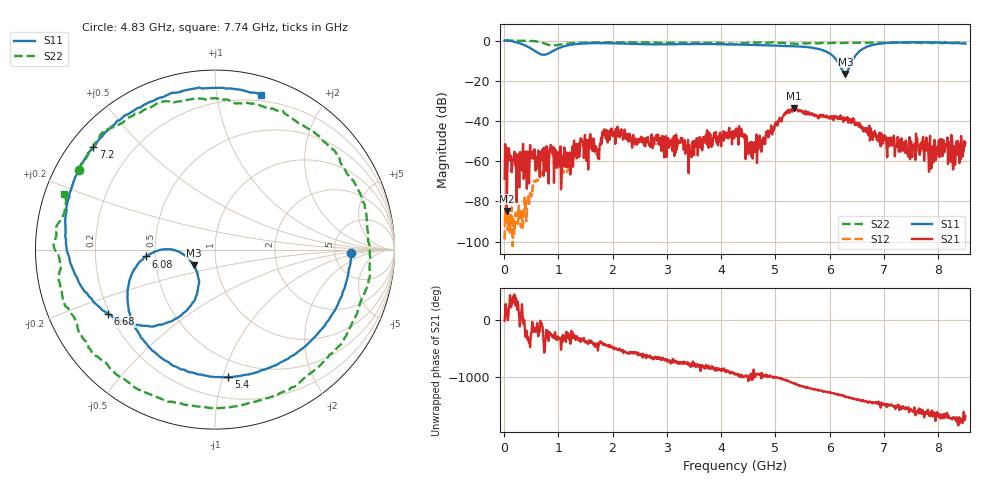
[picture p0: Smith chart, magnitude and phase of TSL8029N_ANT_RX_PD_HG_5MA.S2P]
!Agilent Technologies,E5071C,MY46523237,B.13.01
!Date: Wed Oct 18 11:31:03 2023
!Data & Calibration Information:
!Freq	S11:SOLT2(ON)	S21:SOLT2(ON)	S12:SOLT2(ON)	S22:SOLT2(ON)
!PortZ  Port1:50+j0  Port2:50+j0
!Above PortZ is port z conversion or system Z0 setting when saving the data.
!When reading, reference impedance value at option line is always used.
# Hz S dB R 50
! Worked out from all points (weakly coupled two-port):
!   850 points, 10 MHz to 8.5 GHz, reference 50 ohm
!   highest |S21| = -33.56 dB at 5.34 GHz (marker M1); lowest = -84.8 dB at 50 MHz (marker M2)
!   lowest |S11| = -16.7 dB at 6.29 GHz (marker M3), VSWR 1.34, Z = 38.9 - j6.9 ohm
!   |S11| at or under -10 dB: 6.134 GHz to 6.417 GHz (283.2 MHz wide, 4.51 % of centre)
!   |S22| runs from -2.5 to 0.0 dB; largest |S21 - S12| = 0.0038
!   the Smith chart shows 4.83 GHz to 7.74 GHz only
!   S11 on the Smith chart (normalised r, x): 4.83 GHz: 7.25, -0.74; 5.4 GHz: 0.36, -1.04; 6.08 GHz: 0.44, -0.04; 6.68 GHz: 0.19, -0.27; 7.2 GHz: 0.07, +0.36; 7.74 GHz: 0.14, +1.33
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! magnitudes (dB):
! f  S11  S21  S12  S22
! 10 MHz  0.0  -68.7  -98.9  0.0
! 50 MHz  0.0  -84.8  -86.4  0.0
! 430 MHz  -3.0  -55.1  -80.7  -0.1
! 870 MHz  -5.7  -52.2  -54.2  -2.5
! 1.13 GHz  -2.7  -62.9  -65.7  -1.5
! 1.43 GHz  -1.6  -49.1  -51.9  -1.0
! 2.09 GHz  -1.4  -42.8  -45.4  -0.9
! 2.84 GHz  -1.9  -46.8  -51.3  -1.0
! 3.42 GHz  -1.8  -55.2  -52.0  -1.1
! 4.26 GHz  -2.0  -44.8  -45.4  -1.8
! 4.61 GHz  -2.2  -54.8  -55.4  -1.0
! 4.83 GHz  -2.4  -45.4  -48.2  -1.1
! 5.34 GHz  -2.9  -33.6  -34.3  -1.6
! 5.4 GHz  -2.9  -34.6  -34.5  -1.6
! 5.67 GHz  -3.6  -36.7  -36.6  -1.3
! 6.08 GHz  -8.2  -37.6  -38.3  -1.2
! 6.29 GHz  -16.7  -39.7  -39.0  -1.1
! 6.68 GHz  -3.2  -45.7  -45.0  -1.1
! 7.09 GHz  -1.2  -49.0  -51.2  -1.1
! 7.2 GHz  -1.0  -57.6  -52.2  -1.0
! 7.74 GHz  -0.9  -59.8  -54.4  -1.0
! 8.5 GHz  -1.5  -51.0  -54.5  -1.0
